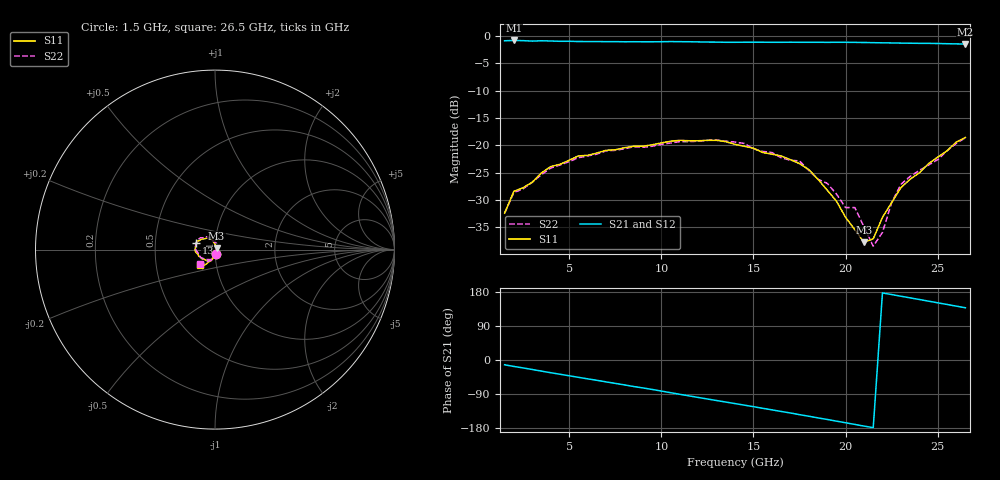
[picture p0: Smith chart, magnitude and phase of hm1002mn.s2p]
! HMMC-1002
! S-PARAMETERS at Minimum Attenuation; V1 = 0V;  V2 = -4V. LAST UPDATED  07-06-99
# GHZ  S  MA  R  50
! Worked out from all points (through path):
!   51 points, 1.5 GHz to 26.5 GHz, reference 50 ohm
!   highest |S21| = -0.86 dB at 2 GHz (marker M1); lowest = -1.5 dB at 26.5 GHz (marker M2)
!   group delay of S21, straight-line fit = 23.2 ps
!   lowest |S11| = -37.7 dB at 21 GHz (marker M3), VSWR 1.03, Z = 50.9 + j0.983 ohm
!   |S11| at or under -10 dB: start of sweep to end of sweep
!   |S22| runs from -38.4 to -18.6 dB; largest |S21 - S12| = 0.0076
!   S11 on the Smith chart (normalised r, x): 1.5 GHz: 1.01, -0.05; 13 GHz: 0.81, +0.06; 26.5 GHz: 0.84, -0.15
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1.5  0.024 -79.9  0.9 -12.6  0.9 -13.0  0.024 -79.4
2  0.038 -80.8  0.906 -17.0  0.906 -17.4  0.037 -80.8
3  0.046 -106.8  0.894 -25.1  0.894 -25.5  0.046 -107.6
4  0.064 -114.1  0.896 -33.6  0.896 -33.9  0.062 -114.6
6  0.081 -138.4  0.885 -49.6  0.885 -49.9  0.08 -139.8
8.5  0.098 -159.3  0.882 -69.9  0.882 -70.1  0.097 -162.5
10  0.105 -169.8  0.882 -81.9  0.882 -82.1  0.102 -174.3
13  0.111 160.9  0.875 -107.0  0.874 -107.0  0.112 155.0
14  0.102 150.8  0.872 -115.0  0.871 -115.0  0.107 145.9
17.5  0.068 117.2  0.872 -144.2  0.872 -144.1  0.072 112.9
18.5  0.049 103.4  0.872 -152.7  0.872 -152.5  0.049 103.2
19  0.039 99.6  0.871 -156.9  0.87 -156.7  0.045 95.3
19.5  0.031 89.7  0.872 -161.3  0.872 -161.0  0.036 75.5
20  0.022 82.2  0.872 -165.6  0.872 -165.4  0.027 71.1
20.5  0.017 75.6  0.87 -170.0  0.87 -169.8  0.027 66.1
21  0.013 48.0  0.868 -174.4  0.867 -174.1  0.018 40.8
21.5  0.014 -21.0  0.865 -178.7  0.864 -178.4  0.012 -16.5
22  0.022 -67.7  0.862 177.0  0.861 177.3  0.016 -73.9
22.5  0.03 -84.7  0.86 172.7  0.86 173.0  0.03 -85.4
23  0.041 -93.2  0.857 168.3  0.857 168.6  0.044 -92.8
24.5  0.068 -110.9  0.852 155.3  0.851 155.8  0.066 -111.1
26.5  0.118 -133.4  0.84 137.8  0.838 138.3  0.117 -135.3
